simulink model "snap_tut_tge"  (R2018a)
settings: Solver=VariableStepDiscrete  StartTime=0.0  StopTime=50000  RelTol=1e-3
undefined symbols (not defined in the file): bad_frame, Bit, Both, bram, c, cnt_rst, core_rst, d, data, data_in, eof, eof_in, Falling, hex2dec, ip, ip_in, led, led_rx, led_tx, led_up, link_up, Location, Lower, Minimum_Area, notused, out, overrun, reg, Rising, ROACH2, sfp, SNAP, tx_full, tx_over, Unsigned, Upper, valid, valid_in, Width, xc7k160t
libraries: xbsIndex_r4 x1201, casper_library_misc x9, xps_library x5
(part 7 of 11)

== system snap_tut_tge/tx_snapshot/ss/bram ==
  addr : Inport
  data_in : Inport  Port=2
  we : Inport  Port=3
  Terminator : Terminator
  Terminator1 : Terminator
  Terminator2 : Terminator
  calc_add : Subsystem  mask{data_width=128, addr_width=12, sample_rate=sample_rate}
      mask prompts: data_width "data width"; addr_width "address width"; sample_rate "sample rate"
  convert_addr : xbsIndex_r4/Convert  gui_display_data_type=Fixed-point  arith_type=Unsigned  n_bits=addr_width  bin_pt=0  float_type=Single  exp_bits=8  fraction_bits=24  quantization=Truncate  overflow=Wrap  en=off  latency=0  pipeline=off  dbl_ovrd=off  block_type=convert
  convert_din1 : xbsIndex_r4/Convert  gui_display_data_type=Fixed-point  arith_type=Unsigned  n_bits=128  bin_pt=0  float_type=Single  exp_bits=8  fraction_bits=24  quantization=Truncate  overflow=Wrap  en=off  latency=0  pipeline=off  dbl_ovrd=off  block_type=convert
  convert_we : xbsIndex_r4/Convert  gui_display_data_type=Fixed-point  arith_type=Unsigned  n_bits=1  bin_pt=0  float_type=Single  exp_bits=8  fraction_bits=24  quantization=Truncate  overflow=Wrap  en=off  latency=0  pipeline=off  dbl_ovrd=off  block_type=convert
  munge_in : Subsystem  AncestorBlock=casper_library_flow_control/munge  mask(munge){divisions=4, div_size=[32 32 32 32], order=[3  2  1  0], arith_type_out=Unsigned, bin_pt_out=0}
      mask prompts: divisions "Number of divisions"; div_size "Division size (bits)"; order "Division packing order"; arith_type_out "Output arithmetic type"; bin_pt_out "Output binary point"
      mask help: Splits an input bus into the specified number of divisions and then recombines them in the order specified (most significant division = 0,least = number divisions-1)
      mask init:
      | munge_init(gcb, ...
      |     'divisions', divisions, ...
      |     'div_size', div_size, ...
      |     'order', order, ...
      |     'arith_type_out', arith_type_out, ...
      |     'bin_pt_out', bin_pt_out);
  munge_out : Subsystem  AncestorBlock=casper_library_flow_control/munge  mask(munge){divisions=4, div_size=[32 32 32 32], order=[3  2  1  0], arith_type_out=Unsigned, bin_pt_out=0}
      mask prompts: divisions "Number of divisions"; div_size "Division size (bits)"; order "Division packing order"; arith_type_out "Output arithmetic type"; bin_pt_out "Output binary point"
      mask help: Splits an input bus into the specified number of divisions and then recombines them in the order specified (most significant division = 0,least = number divisions-1)
      mask init:
      | munge_init(gcb, ...
      |     'divisions', divisions, ...
      |     'div_size', div_size, ...
      |     'order', order, ...
      |     'arith_type_out', arith_type_out, ...
      |     'bin_pt_out', bin_pt_out);
  sim_mem : Subsystem  mask{arith_type=Unsigned, addr_width=12, data_width=128, data_bin_pt=0, init_vals=[0     1     2     3     4     5     6     7     8     9    10    11    12    13    14    15    16    17    18    19    20    21    22    23    24    25    26    27    28    29    30    31    32    33    34    35    36    37    38    39    40    41    42    43    44    45    46    47    48    49    50    51    52    53    54    55    56    57    58    59    60    61    62    63    64    65    66  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, sample_rate=1, csp_latency=1}
      mask prompts: arith_type "Output Data Type"; addr_width "Address width"; data_width "Data width"; data_bin_pt "Data Binary Point"; init_vals "Initial values"; sample_rate "Sample rate"; csp_latency "Latency"
      mask init:
      | % set_param([gcb, '/data_to_xilinx'], 'arith_type', arith_type)
      | % set_param([gcb, '/data_to_xilinx'], 'n_bits', get_param(gcb, 'data_width'))
  snap_tut_tge_tx_snapshot_ss_bram_addr : xbsIndex_r4/Gateway Out  inherit_from_input=off  hdl_port=on  rows=1  columns=1  UseAsDAC=off  DACChannel='1'  interface=None  automatic_assignment=on  address_offset=hex2dec('00')  intf_name=''  intf_description=''  timing_constraint=None  locs_specified=off  LOCs={'A5','B9','A9','C1','A3','G6','E9','A6','A7','A8','B8','B1','B3','D9','B5','B4','B6','C2'}  io_standard={}  block_type=gatewayout
  snap_tut_tge_tx_snapshot_ss_bram_data_in : xbsIndex_r4/Gateway Out  inherit_from_input=off  hdl_port=on  rows=1  columns=1  UseAsDAC=off  DACChannel='1'  interface=None  automatic_assignment=on  address_offset=hex2dec('00')  intf_name=''  intf_description=''  timing_constraint=None  locs_specified=off  LOCs={'B21','B22','A22','B23','B19','C19','A20','A21','A23','B24','A24','A25','E18','D18','C18','B18'}  io_standard={}  block_type=gatewayout
  snap_tut_tge_tx_snapshot_ss_bram_data_out : xbsIndex_r4/Gateway In  gui_display_data_type=Fixed-point  arith_type=Unsigned  n_bits=128  bin_pt=0  preci_type=Single  exp_width=8  frac_width=24  rows=1  columns=1  quantization=Truncate  overflow=Wrap  period=sample_rate  UseAsADC=off  ADCChannel='1'  interface=None  automatic_assignment=on  address_offset=hex2dec('00')  intf_name=''  intf_description=''  default_value=0  timing_constraint=None  locs_specified=off  LOCs={}  io_standard={}  inherit_from_input=off  hdl_port=on  dbl_ovrd=off  block_type=gatewayin
  snap_tut_tge_tx_snapshot_ss_bram_we : xbsIndex_r4/Gateway Out  inherit_from_input=off  hdl_port=on  rows=1  columns=1  UseAsDAC=off  DACChannel='1'  interface=None  automatic_assignment=on  address_offset=hex2dec('00')  intf_name=''  intf_description=''  timing_constraint=None  locs_specified=off  LOCs={'A14'}  io_standard={}  block_type=gatewayout
  data_out : Outport
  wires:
  munge_in/1(dout) -> convert_din1/1, sim_mem/2(data)
  we/1 -> convert_we/1, sim_mem/3(we)
  addr/1 -> calc_add/1(in)
  convert_we/1 -> snap_tut_tge_tx_snapshot_ss_bram_we/1
  snap_tut_tge_tx_snapshot_ss_bram_addr/1 -> Terminator/1
  snap_tut_tge_tx_snapshot_ss_bram_data_in/1 -> Terminator1/1
  snap_tut_tge_tx_snapshot_ss_bram_we/1 -> Terminator2/1
  calc_add/1(out) -> convert_addr/1, sim_mem/1(addr)
  data_in/1 -> munge_in/1(din)
  convert_din1/1 -> snap_tut_tge_tx_snapshot_ss_bram_data_in/1
  convert_addr/1 -> snap_tut_tge_tx_snapshot_ss_bram_addr/1
  snap_tut_tge_tx_snapshot_ss_bram_data_out/1 -> munge_out/1(din)
  sim_mem/1(data_out) -> snap_tut_tge_tx_snapshot_ss_bram_data_out/1
  munge_out/1(dout) -> data_out/1

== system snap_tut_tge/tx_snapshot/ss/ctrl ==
  convert1_1 : DataTypeConversion  OutDataTypeStr=fixdt('ufix32_En0')
  convert2_1 : DataTypeConversion  OutDataTypeStr=fixdt('ufix32_En0')  ConvertRealWorld=Stored Integer (SI)
  gain_1 : Gain
  io_delay : xbsIndex_r4/Delay  rst=off  infoeditControl=Selection of Reset will increase slice count due to use of real FFs and instead of SRLs  en=off  latency=0  reg_retiming=on  dbl_ovrd=off  block_type=delay
  reint1 : xbsIndex_r4/Reinterpret  force_arith_type=on  arith_type=Unsigned  force_bin_pt=on  bin_pt=0  block_type=reinterpret
  sim_1 : Constant  Value=0
  slice_reg : xbsIndex_r4/Slice  nbits=32  boolean_output=off  mode=Lower Bit Location + Width  bit1=0  base1=MSB of Input  bit0=0  base0=LSB of Input  dbl_ovrd=off  block_type=slice
  snap_tut_tge_tx_snapshot_ss_ctrl_user_data_out : xbsIndex_r4/Gateway In  gui_display_data_type=Fixed-point  arith_type=Unsigned  n_bits=32  bin_pt=0  preci_type=Single  exp_width=8  frac_width=24  rows=1  columns=1  quantization="Round  (unbiased: +/- Inf)"  overflow=Saturate  period=1  UseAsADC=off  ADCChannel='1'  interface=None  automatic_assignment=on  address_offset=hex2dec('00')  intf_name=''  intf_description=''  default_value=0  timing_constraint=None  locs_specified=off  LOCs={}  io_standard={}  inherit_from_input=off  hdl_port=on  dbl_ovrd=off  block_type=gatewayin
  in_reg : Outport
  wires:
  snap_tut_tge_tx_snapshot_ss_ctrl_user_data_out/1 -> io_delay/1
  sim_1/1 -> convert1_1/1
  convert1_1/1 -> convert2_1/1
  convert2_1/1 -> gain_1/1
  gain_1/1 -> snap_tut_tge_tx_snapshot_ss_ctrl_user_data_out/1
  io_delay/1 -> slice_reg/1
  slice_reg/1 -> reint1/1
  reint1/1 -> in_reg/1

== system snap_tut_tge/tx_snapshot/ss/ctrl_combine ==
  in1 : Inport
  in2 : Inport  Port=2
  in3 : Inport  Port=3
  in4 : Inport  Port=4
  concatenate : xbsIndex_r4/Concat  num_inputs=4  dbl_ovrd=off  block_type=concat
  reinterpret{1..4} (4 alike) : xbsIndex_r4/Reinterpret  force_arith_type=on  arith_type=Unsigned  force_bin_pt=on  bin_pt=0  block_type=reinterpret
  bus_out : Outport
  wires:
  concatenate/1 -> bus_out/1
  in1/1 -> reinterpret1/1
  reinterpret1/1 -> concatenate/1
  in2/1 -> reinterpret2/1
  reinterpret2/1 -> concatenate/2
  in3/1 -> reinterpret3/1
  reinterpret3/1 -> concatenate/3
  in4/1 -> reinterpret4/1
  reinterpret4/1 -> concatenate/4

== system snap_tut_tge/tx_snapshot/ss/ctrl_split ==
  bus_in : Inport
  reinterpret2 : xbsIndex_r4/Reinterpret  force_arith_type=on  arith_type=Unsigned  force_bin_pt=on  bin_pt=0  block_type=reinterpret
  reinterpret4 : xbsIndex_r4/Reinterpret  force_arith_type=on  arith_type=Unsigned  force_bin_pt=on  bin_pt=0  block_type=reinterpret
  slice1 : xbsIndex_r4/Slice  nbits=1  boolean_output=on  mode=Upper Bit Location + Width  bit1=-31  base1=MSB of Input  bit0=0  base0=LSB of Input  dbl_ovrd=off  block_type=slice
  slice2 : xbsIndex_r4/Slice  nbits=2  boolean_output=off  mode=Upper Bit Location + Width  bit1=-29  base1=MSB of Input  bit0=0  base0=LSB of Input  dbl_ovrd=off  block_type=slice
  slice3 : xbsIndex_r4/Slice  nbits=1  boolean_output=on  mode=Upper Bit Location + Width  bit1=-28  base1=MSB of Input  bit0=0  base0=LSB of Input  dbl_ovrd=off  block_type=slice
  slice4 : xbsIndex_r4/Slice  nbits=28  boolean_output=off  mode=Upper Bit Location + Width  bit1=0  base1=MSB of Input  bit0=0  base0=LSB of Input  dbl_ovrd=off  block_type=slice
  msb_out4 : Outport
  out3 : Outport  Port=2
  out2 : Outport  Port=3
  lsb_out1 : Outport  Port=4
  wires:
  bus_in/1 -> slice4/1, slice3/1, slice2/1, slice1/1
  slice4/1 -> reinterpret4/1
  reinterpret4/1 -> msb_out4/1
  slice3/1 -> out3/1
  slice2/1 -> reinterpret2/1
  reinterpret2/1 -> out2/1
  slice1/1 -> lsb_out1/1

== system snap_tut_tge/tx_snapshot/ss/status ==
  out_reg : Inport
  assert_reg : xbsIndex_r4/Assert  assert_type=on  type_source=Explicitly  gui_display_data_type=Fixed-point  arith_type=Unsigned  n_bits=32  bin_pt=0  preci_type=Single  exp_width=8  frac_width=24  assert_rate=off  rate_source=Explicitly  period=1  output_port=on  block_type=assert
  cast_gw : xbsIndex_r4/Convert  gui_display_data_type=Fixed-point  arith_type=Unsigned  n_bits=32  bin_pt=0  float_type=Single  exp_bits=8  fraction_bits=24  quantization=Truncate  overflow=Wrap  en=off  latency=1  pipeline=off  dbl_ovrd=off  block_type=convert
  io_delay : xbsIndex_r4/Delay  rst=off  infoeditControl=Selection of Reset will increase slice count due to use of real FFs and instead of SRLs  en=off  latency=0  reg_retiming=on  dbl_ovrd=off  block_type=delay
  reint1 : xbsIndex_r4/Reinterpret  force_arith_type=on  arith_type=Unsigned  force_bin_pt=on  bin_pt=0  block_type=reinterpret
  sim_out : Terminator
  snap_tut_tge_tx_snapshot_ss_status_user_data_in : xbsIndex_r4/Gateway Out  inherit_from_input=off  hdl_port=on  rows=1  columns=1  UseAsDAC=off  DACChannel='1'  interface=None  automatic_assignment=on  address_offset=hex2dec('00')  intf_name=''  intf_description=''  timing_constraint=None  locs_specified=off  LOCs={}  io_standard={}  block_type=gatewayout
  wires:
  io_delay/1 -> cast_gw/1
  cast_gw/1 -> snap_tut_tge_tx_snapshot_ss_status_user_data_in/1
  snap_tut_tge_tx_snapshot_ss_status_user_data_in/1 -> sim_out/1
  out_reg/1 -> assert_reg/1
  assert_reg/1 -> reint1/1
  reint1/1 -> io_delay/1

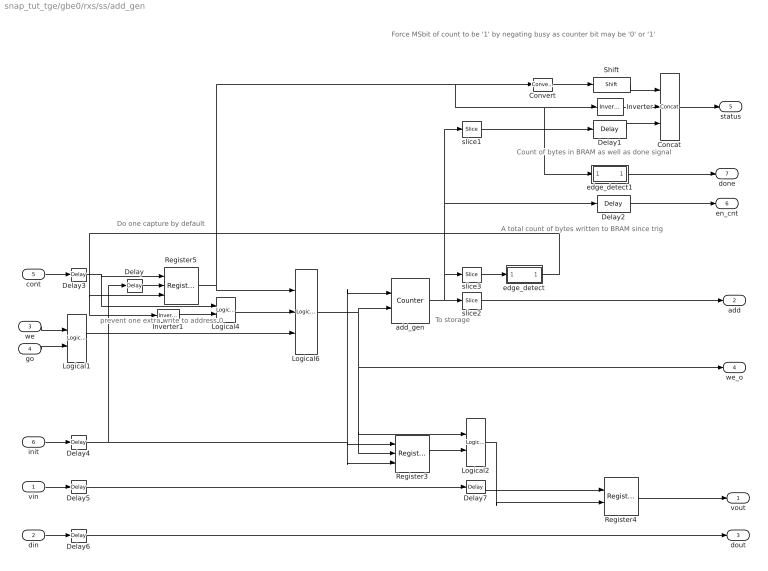
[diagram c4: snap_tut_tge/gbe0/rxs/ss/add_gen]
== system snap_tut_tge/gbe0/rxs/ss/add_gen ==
  note: Force MSbit of count to be '1' by negating busy as counter bit may be '0' or '1'
  note: A total count of bytes written to BRAM since trig
  note: Count of bytes in BRAM as well as done signal
  note: Do one capture by default
  note: prevent one extra write to address 0
  note: To storage
  vin : Inport
  din : Inport  Port=2
  we : Inport  Port=3
  go : Inport  Port=4
  cont : Inport  Port=5
  init : Inport  Port=6
  Concat : xbsIndex_r4/Concat  num_inputs=3  dbl_ovrd=off  block_type=concat
  Convert : xbsIndex_r4/Convert  gui_display_data_type=Fixed-point  arith_type=Unsigned  n_bits=32-nsamples-log2(increment)-1  bin_pt=0  float_type=Single  exp_bits=8  fraction_bits=24  quantization=Truncate  overflow=Wrap  en=off  latency=0  pipeline=off  dbl_ovrd=off  block_type=convert
  Delay{,3..6} (5 alike) : xbsIndex_r4/Delay  rst=off  infoeditControl=Selection of Reset will increase slice count due to use of real FFs and instead of SRLs  en=off  latency=1  reg_retiming=on  dbl_ovrd=off  block_type=delay
  Delay1 : xbsIndex_r4/Delay  rst=off  infoeditControl=Selection of Reset will increase slice count due to use of real FFs and instead of SRLs  en=off  latency=1  reg_retiming=off  dbl_ovrd=off  block_type=delay
  Delay2 : xbsIndex_r4/Delay  rst=off  infoeditControl=Selection of Reset will increase slice count due to use of real FFs and instead of SRLs  en=off  latency=1  reg_retiming=off  dbl_ovrd=off  block_type=delay
  Delay7 : xbsIndex_r4/Delay  rst=off  infoeditControl=Selection of Reset will increase slice count due to use of real FFs and instead of SRLs  en=off  latency=1  reg_retiming=off  dbl_ovrd=off  block_type=delay
  Inverter : xbsIndex_r4/Inverter  en=off  latency=1  dbl_ovrd=off  block_type=inv
  Inverter1 : xbsIndex_r4/Inverter  en=off  latency=0  dbl_ovrd=off  block_type=inv
  Logical1 : xbsIndex_r4/Logical  logical_function=AND  inputs=2  en=off  latency=1  precision=Full  arith_type=Unsigned  n_bits=8  bin_pt=2  align_bp=on  dbl_ovrd=off  block_type=logical
  Logical2 : xbsIndex_r4/Logical  logical_function=AND  inputs=2  en=off  latency=1  precision=Full  arith_type=Unsigned  n_bits=8  bin_pt=2  align_bp=on  dbl_ovrd=off  block_type=logical
  Logical4 : xbsIndex_r4/Logical  logical_function=OR  inputs=2  en=off  latency=0  precision=Full  arith_type=Unsigned  n_bits=8  bin_pt=2  align_bp=on  dbl_ovrd=off  block_type=logical
  Logical6 : xbsIndex_r4/Logical  logical_function=AND  inputs=3  en=off  latency=0  precision=Full  arith_type=Unsigned  n_bits=8  bin_pt=2  align_bp=on  dbl_ovrd=off  block_type=logical
  Register3 : xbsIndex_r4/Register  init=0  rst=on  en=on  dbl_ovrd=off  block_type=register
  Register4 : xbsIndex_r4/Register  init=0  rst=off  en=on  dbl_ovrd=off  block_type=register
  Register5 : xbsIndex_r4/Register  init=1  rst=on  en=on  dbl_ovrd=off  block_type=register
  Shift : xbsIndex_r4/Shift  shift_dir=Left  shift_bits=32-nsamples-log2(increment)-1-1  en=off  latency=1  precision=Full  arith_type="Signed  (2's comp)"  n_bits=16  bin_pt=14  quantization=Truncate  overflow=Wrap  dbl_ovrd=off  block_type=shift
  add_gen : xbsIndex_r4/Counter  cnt_type=Free Running  cnt_to=1  operation=Up  start_count=0  cnt_by_val=increment  arith_type=Unsigned  n_bits=counter_size  bin_pt=0  load_pin=off  rst=on  en=on  explicit_period=on  period=1  use_behavioral_HDL=off  implementation=DSP48  use_rpm=on  dbl_ovrd=off  block_type=counter
  edge_detect : Subsystem  AncestorBlock=casper_library_misc/edge_detect  mask(edge_detect){edge=Both, polarity=Active High, x_in=[0 0.08 0.08 0.16 0.16 0.24 0.24 0.32 0.32 0.4], y_in=[-1 -1  1  1  1  1 -1 -1 -1 -1], x_out=[0.6 0.68 0.68 0.76 0.76 0.84 0.84 0.92 0.92 1], y_out=[-1 -1  1  1 -1 -1  1  1 -1 -1]}
      mask prompts: edge "Edge Type"; polarity "Output Polarity"; x_in "Input X Positions"; y_in "Input Y Positions"; x_out "Output X Positions"; y_out "Output Y Positions"
      mask help: Output is active for one-cycle after each edge of the specified type (i.e. rising, falling or both).
      mask init:
      | edge_detect_init(gcb,...
      |     'edge',edge,...
      |     'polarity',polarity,...
      |     'x_in',x_in,...
      |     'x_out',x_out,...
      |     'y_in',y_in,...
      |     'y_out',y_out);
      | 
      | x_in_num=str2num(getfield(getfield(get_param(gcb,'UserData'),'parameters'),'x_in'));
      | x_out_num=str2num(getfield(getfield(get_param(gcb,'UserData'),'parameters'),'x_out'));
      | y_in_num=str2num(getfield(getfield(get_param(gcb,'UserData'),'parameters'),'y_in'));
      | y_out_num=str2num(getfield(getfield(get_param(gcb,'UserData'),'parameters'),'y_out'));
  edge_detect1 : Subsystem  AncestorBlock=casper_library_scopes/snapshot/add_gen/edge_detect  mask(edge_detect){edge=Both, polarity=Active High, x_in=[0 0.08 0.08 0.16 0.16 0.24 0.24 0.32 0.32 0.4], y_in=[-1 -1  1  1  1  1 -1 -1 -1 -1], x_out=[0.6 0.68 0.68 0.76 0.76 0.84 0.84 0.92 0.92 1], y_out=[-1 -1  1  1 -1 -1  1  1 -1 -1]}
      mask prompts: edge "Edge Type"; polarity "Output Polarity"; x_in "Input X Positions"; y_in "Input Y Positions"; x_out "Output X Positions"; y_out "Output Y Positions"
      mask help: Output is active for one-cycle after each edge of the specified type (i.e. rising, falling or both).
      mask init:
      | edge_detect_init(gcb,...
      |     'edge',edge,...
      |     'polarity',polarity,...
      |     'x_in',x_in,...
      |     'x_out',x_out,...
      |     'y_in',y_in,...
      |     'y_out',y_out);
      | 
      | x_in_num=str2num(getfield(getfield(get_param(gcb,'UserData'),'parameters'),'x_in'));
      | x_out_num=str2num(getfield(getfield(get_param(gcb,'UserData'),'parameters'),'x_out'));
      | y_in_num=str2num(getfield(getfield(get_param(gcb,'UserData'),'parameters'),'y_in'));
      | y_out_num=str2num(getfield(getfield(get_param(gcb,'UserData'),'parameters'),'y_out'));
  slice1 : xbsIndex_r4/Slice  nbits=nsamples+log2(increment)  boolean_output=off  mode=Lower Bit Location + Width  bit1=0  base1=LSB of Input  bit0=0  base0=LSB of Input  dbl_ovrd=off  block_type=slice
  slice2 : xbsIndex_r4/Slice  nbits=nsamples-burst_size  boolean_output=off  mode=Lower Bit Location + Width  bit1=0  base1=LSB of Input  bit0=log2(increment)+burst_size  base0=LSB of Input  dbl_ovrd=off  block_type=slice
  slice3 : xbsIndex_r4/Slice  nbits=1  boolean_output=on  mode=Lower Bit Location + Width  bit1=0  base1=MSB of Input  bit0=nsamples + log2(increment)  base0=LSB of Input  dbl_ovrd=off  block_type=slice
  vout : Outport
  add : Outport  Port=2
  dout : Outport  Port=3
  we_o : Outport  Port=4
  status : Outport  Port=5
  en_cnt : Outport  Port=6
  done : Outport  Port=7
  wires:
  Delay6/1 -> dout/1
  Delay5/1 -> Delay7/1
  Delay4/1 -> Delay/1, Register3/1, Register3/3, add_gen/1
  Delay3/1 -> Register5/1, Logical4/1
  Delay7/1 -> Register4/1
  Logical1/1 -> Logical6/3
  go/1 -> Logical1/2
  we/1 -> Logical1/1
  Logical4/1 -> Logical6/2
  Inverter/1 -> Concat/2
  slice1/1 -> Delay1/1
  Delay1/1 -> Concat/3
  din/1 -> Delay6/1
  Delay2/1 -> en_cnt/1
  slice2/1 -> add/1
  Convert/1 -> Shift/1
  Concat/1 -> status/1
  Logical6/1 -> add_gen/2, Register3/2, Logical2/1, we_o/1
  init/1 -> Delay4/1
  slice3/1 -> edge_detect/1(in)
  Register5/1 -> Logical6/1, edge_detect1/1(in), Inverter/1, Convert/1
  add_gen/1 -> slice3/1, Delay2/1, slice1/1, slice2/1
  vin/1 -> Delay5/1
  Register3/1 -> Logical2/2
  Logical2/1 -> Register4/2
  Register4/1 -> vout/1
  edge_detect/1(out) -> Register5/3, Inverter1/1
  cont/1 -> Delay3/1
  Inverter1/1 -> Logical4/2
  Delay/1 -> Register5/2
  Shift/1 -> Concat/1
  edge_detect1/1(out) -> done/1

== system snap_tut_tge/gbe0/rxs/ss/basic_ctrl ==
  vin : Inport
  din : Inport  Port=2
  we : Inport  Port=3
  trig : Inport  Port=4
  ctrl : Inport  Port=5
  stopi : Inport  Port=6
  Constant : xbsIndex_r4/Constant  const=1  gui_display_data_type=Fixed-point  arith_type=Boolean  n_bits=16  bin_pt=14  preci_type=Single  exp_width=8  frac_width=24  explicit_period=on  period=1  equ=P=C  opselect=C  inp2=PCIN>>17  opr=+  inp1=P  carry=CIN  dbl_ovrd=off  block_type=constant
  Constant1 : xbsIndex_r4/Constant  const=1  gui_display_data_type=Fixed-point  arith_type=Boolean  n_bits=1  bin_pt=0  preci_type=Single  exp_width=8  frac_width=24  explicit_period=on  period=1  equ=P=C  opselect=C  inp2=PCIN>>17  opr=+  inp1=P  carry=CIN  dbl_ovrd=off  block_type=constant
  Constant2 : xbsIndex_r4/Constant  const=1  gui_display_data_type=Fixed-point  arith_type=Boolean  n_bits=1  bin_pt=0  preci_type=Single  exp_width=8  frac_width=24  explicit_period=on  period=1  equ=P=C  opselect=C  inp2=PCIN>>17  opr=+  inp1=P  carry=CIN  dbl_ovrd=off  block_type=constant
  Delay1 : xbsIndex_r4/Delay  rst=off  infoeditControl=Selection of Reset will increase slice count due to use of real FFs and instead of SRLs  en=off  latency=1  reg_retiming=off  dbl_ovrd=off  block_type=delay
  Delay2 : xbsIndex_r4/Delay  rst=off  infoeditControl=Selection of Reset will increase slice count due to use of real FFs and instead of SRLs  en=off  latency=1  reg_retiming=off  dbl_ovrd=off  block_type=delay
  Delay3 : xbsIndex_r4/Delay  rst=off  infoeditControl=Selection of Reset will increase slice count due to use of real FFs and instead of SRLs  en=off  latency=1  reg_retiming=off  dbl_ovrd=off  block_type=delay
  Inverter : xbsIndex_r4/Inverter  en=off  latency=0  dbl_ovrd=off  block_type=inv
  Logical : xbsIndex_r4/Logical  logical_function=AND  inputs=2  en=off  latency=0  precision=Full  arith_type=Unsigned  n_bits=16  bin_pt=0  align_bp=on  dbl_ovrd=off  block_type=logical
  Mux1 : xbsIndex_r4/Mux  inputs=2  en=off  latency=0  precision=Full  arith_type="Signed  (2's comp)"  n_bits=8  bin_pt=2  quantization=Truncate  overflow=Wrap  dbl_ovrd=off  block_type=mux
  Mux2 : xbsIndex_r4/Mux  inputs=2  en=off  latency=0  precision=Full  arith_type="Signed  (2's comp)"  n_bits=8  bin_pt=2  quantization=Truncate  overflow=Wrap  dbl_ovrd=off  block_type=mux
  Register1 : xbsIndex_r4/Register  init=0  rst=on  en=on  dbl_ovrd=off  block_type=register
  Register6 : xbsIndex_r4/Register  init=0  rst=on  en=on  dbl_ovrd=off  block_type=register
  dram_munge : Subsystem  mask{dram=off, data_width=data_width}
      mask prompts: data_width "data width"
      mask init:
      | set_param(gcb,'LinkStatus','inactive');
      | if strcmp(dram,'on'),
      |     set_param([gcb,'/dram'], 'const', '1');
      | else,
      |     set_param([gcb,'/dram'], 'const', '0');
      | end
      | set_param([gcb,'/data_choice'], ...
      |         'precision', 'User Defined', ...
      |         'arith_type', 'Unsigned', ...
      |         'n_bits', num2str(data_width), 'bin_pt', '0', ...
      |         'quantization', 'Truncate', ...
      |         'overflow', 'Wrap');
  edge_detect : casper_library_misc/edge_detect  edge=Rising  polarity=Active High  x_in=[0 0.08 0.08 0.16 0.16 0.24 0.24 0.32 0.32 0.4]  y_in="[-1 -1  1  1  1  1  1  1  1  1]"  x_out=[0.6 0.68 0.68 0.76 0.76 0.84 0.84 0.92 0.92 1]  y_out="[-1 -1  1  1 -1 -1 -1 -1 -1 -1]"
      link override Delay: sg_icon_stat=45,16,1,1,white,blue,0,07b98262,right,,[ ],[ ]  sg_mask_display=fprintf('','COMMENT: begin icon graphics'); patch([0 45 45 0 0 ],[0 0 16 16 0 ],[0.77 0.82 0.91 ]); plot([0 45 45 0 0 ],[0 0 16 16 0 ]); patch([17.55 20.44 22.44 24.44 26.44 22.44 19.55 17.55 ],[10.22 10.22 12.22 10.22 12.22 12.22 12.22 10.22 ],[1 1 1 ]); patch([19.55 22.44 20.44 17.55 19.55 ],[8.22 8.22 10.22 10.22 8.22 ],[0.931 0.946 0.973 ]); patch([17.55 20.44 22.44 19.55 17.55 ],[6.22 6.22 8.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
      link override Inverter: sg_icon_stat=45,16,1,1,white,blue,0,267846e5,right,,[ ],[ ]  sg_mask_display=fprintf('','COMMENT: begin icon graphics'); patch([0 45 45 0 0 ],[0 0 16 16 0 ],[0.77 0.82 0.91 ]); plot([0 45 45 0 0 ],[0 0 16 16 0 ]); patch([17.55 20.44 22.44 24.44 26.44 22.44 19.55 17.55 ],[10.22 10.22 12.22 10.22 12.22 12.22 12.22 10.22 ],[1 1 1 ]); patch([19.55 22.44 20.44 17.55 19.55 ],[8.22 8.22 10.22 10.22 8.22 ],[0.931 0.946 0.973 ]); patch([17.55 20.44 22.44 19.55 17.55 ],[6.22 6.22 8.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
      link override edge_op: sg_icon_stat=45,44,2,1,white,blue,0,affe8783,right,,[ ],[ ]  sg_mask_display=fprintf('','COMMENT: begin icon graphics'); patch([0 45 45 0 0 ],[0 0 44 44 0 ],[0.77 0.82 0.91 ]); plot([0 45 45 0 0 ],[0 0 44 44 0 ]); patch([8.65 17.32 23.32 29.32 35.32 23.32 14.65 8.65 ],[28.66 28.66 34.66 28.66 34.66 34.66 34.66 28.66 ],[1 1 1 ]); patch([14.65 23.32 17.32 8.65 14.65 ],[22.66 22.66 28.66 28.66 22.66 ],[0.931 0.946 0.973 ]); patch([8.65 17.32 23.32 14.65 8.65 ],[16.66 16.66 22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
  enable : xbsIndex_r4/Slice  nbits=1  boolean_output=on  mode=Lower Bit Location + Width  bit1=0  base1=LSB of Input  bit0=0  base0=LSB of Input  dbl_ovrd=off  block_type=slice
  trig_src : xbsIndex_r4/Slice  nbits=1  boolean_output=on  mode=Lower Bit Location + Width  bit1=0  base1=LSB of Input  bit0=1  base0=LSB of Input  dbl_ovrd=off  block_type=slice
  valid_src : xbsIndex_r4/Slice  nbits=1  boolean_output=on  mode=Lower Bit Location + Width  bit1=0  base1=LSB of Input  bit0=2  base0=LSB of Input  dbl_ovrd=off  block_type=slice
  vout : Outport
  dout : Outport  Port=2
  we_o : Outport  Port=3
  go : Outport  Port=4
  stop : Outport  Port=5
  init : Outport  Port=6
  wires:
  Delay1/1 -> edge_detect/1
  Delay3/1 -> Mux1/1
  Delay2/1 -> Mux2/1
  dram_munge/1(vout) -> vout/1
  vin/1 -> dram_munge/1(vin)
  dram_munge/3(we_o) -> we_o/1
  dram_munge/2(dout) -> dout/1
  din/1 -> dram_munge/2(din)
  Inverter/1 -> Logical/2
  Mux2/1 -> Logical/1, Register6/1
  Register6/1 -> go/1
  trig/1 -> Mux2/2
  Mux1/1 -> dram_munge/3(we)
  we/1 -> Mux1/2
  ctrl/1 -> enable/1, valid_src/1, trig_src/1
  edge_detect/1 -> Inverter/1, Register1/3, dram_munge/4(init), Register6/2, init/1
  enable/1 -> Delay1/1
  Constant1/1 -> Mux2/3
  Constant2/1 -> Mux1/3
  trig_src/1 -> Delay2/1
  valid_src/1 -> Delay3/1
  Constant/1 -> Register1/1
  Register1/1 -> Register6/3
  Logical/1 -> Register1/2
  stopi/1 -> stop/1

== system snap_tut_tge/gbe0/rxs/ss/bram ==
  addr : Inport
  data_in : Inport  Port=2
  we : Inport  Port=3
  Terminator : Terminator
  Terminator1 : Terminator
  Terminator2 : Terminator
  calc_add : Subsystem  mask{data_width=128, addr_width=13, sample_rate=sample_rate}
      mask prompts: data_width "data width"; addr_width "address width"; sample_rate "sample rate"
  convert_addr : xbsIndex_r4/Convert  gui_display_data_type=Fixed-point  arith_type=Unsigned  n_bits=addr_width  bin_pt=0  float_type=Single  exp_bits=8  fraction_bits=24  quantization=Truncate  overflow=Wrap  en=off  latency=0  pipeline=off  dbl_ovrd=off  block_type=convert
  convert_din1 : xbsIndex_r4/Convert  gui_display_data_type=Fixed-point  arith_type=Unsigned  n_bits=128  bin_pt=0  float_type=Single  exp_bits=8  fraction_bits=24  quantization=Truncate  overflow=Wrap  en=off  latency=0  pipeline=off  dbl_ovrd=off  block_type=convert
  convert_we : xbsIndex_r4/Convert  gui_display_data_type=Fixed-point  arith_type=Unsigned  n_bits=1  bin_pt=0  float_type=Single  exp_bits=8  fraction_bits=24  quantization=Truncate  overflow=Wrap  en=off  latency=0  pipeline=off  dbl_ovrd=off  block_type=convert
  munge_in : Subsystem  AncestorBlock=casper_library_flow_control/munge  mask(munge){divisions=4, div_size=[32 32 32 32], order=[3  2  1  0], arith_type_out=Unsigned, bin_pt_out=0}
      mask prompts: divisions "Number of divisions"; div_size "Division size (bits)"; order "Division packing order"; arith_type_out "Output arithmetic type"; bin_pt_out "Output binary point"
      mask help: Splits an input bus into the specified number of divisions and then recombines them in the order specified (most significant division = 0,least = number divisions-1)
      mask init:
      | munge_init(gcb, ...
      |     'divisions', divisions, ...
      |     'div_size', div_size, ...
      |     'order', order, ...
      |     'arith_type_out', arith_type_out, ...
      |     'bin_pt_out', bin_pt_out);
  munge_out : Subsystem  AncestorBlock=casper_library_flow_control/munge  mask(munge){divisions=4, div_size=[32 32 32 32], order=[3  2  1  0], arith_type_out=Unsigned, bin_pt_out=0}
      mask prompts: divisions "Number of divisions"; div_size "Division size (bits)"; order "Division packing order"; arith_type_out "Output arithmetic type"; bin_pt_out "Output binary point"
      mask help: Splits an input bus into the specified number of divisions and then recombines them in the order specified (most significant division = 0,least = number divisions-1)
      mask init:
      | munge_init(gcb, ...
      |     'divisions', divisions, ...
      |     'div_size', div_size, ...
      |     'order', order, ...
      |     'arith_type_out', arith_type_out, ...
      |     'bin_pt_out', bin_pt_out);
  sim_mem : Subsystem  mask{arith_type=Unsigned, addr_width=13, data_width=128, data_bin_pt=0, init_vals=[0     1     2     3     4     5     6     7     8     9    10    11    12    13    14    15    16    17    18    19    20    21    22    23    24    25    26    27    28    29    30    31    32    33    34    35    36    37    38    39    40    41    42    43    44    45    46    47    48    49    50    51    52    53    54    55    56    57    58    59    60    61    62    63    64    65    66  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, sample_rate=1, csp_latency=1}
      mask prompts: arith_type "Output Data Type"; addr_width "Address width"; data_width "Data width"; data_bin_pt "Data Binary Point"; init_vals "Initial values"; sample_rate "Sample rate"; csp_latency "Latency"
      mask init:
      | % set_param([gcb, '/data_to_xilinx'], 'arith_type', arith_type)
      | % set_param([gcb, '/data_to_xilinx'], 'n_bits', get_param(gcb, 'data_width'))
  snap_tut_tge_gbe0_rxs_ss_bram_addr : xbsIndex_r4/Gateway Out  inherit_from_input=off  hdl_port=on  rows=1  columns=1  UseAsDAC=off  DACChannel='1'  interface=None  automatic_assignment=on  address_offset=hex2dec('00')  intf_name=''  intf_description=''  timing_constraint=None  locs_specified=off  LOCs={'A5','B9','A9','C1','A3','G6','E9','A6','A7','A8','B8','B1','B3','D9','B5','B4','B6','C2'}  io_standard={}  block_type=gatewayout
  snap_tut_tge_gbe0_rxs_ss_bram_data_in : xbsIndex_r4/Gateway Out  inherit_from_input=off  hdl_port=on  rows=1  columns=1  UseAsDAC=off  DACChannel='1'  interface=None  automatic_assignment=on  address_offset=hex2dec('00')  intf_name=''  intf_description=''  timing_constraint=None  locs_specified=off  LOCs={'B21','B22','A22','B23','B19','C19','A20','A21','A23','B24','A24','A25','E18','D18','C18','B18'}  io_standard={}  block_type=gatewayout
  snap_tut_tge_gbe0_rxs_ss_bram_data_out : xbsIndex_r4/Gateway In  gui_display_data_type=Fixed-point  arith_type=Unsigned  n_bits=128  bin_pt=0  preci_type=Single  exp_width=8  frac_width=24  rows=1  columns=1  quantization=Truncate  overflow=Wrap  period=sample_rate  UseAsADC=off  ADCChannel='1'  interface=None  automatic_assignment=on  address_offset=hex2dec('00')  intf_name=''  intf_description=''  default_value=0  timing_constraint=None  locs_specified=off  LOCs={}  io_standard={}  inherit_from_input=off  hdl_port=on  dbl_ovrd=off  block_type=gatewayin
  snap_tut_tge_gbe0_rxs_ss_bram_we : xbsIndex_r4/Gateway Out  inherit_from_input=off  hdl_port=on  rows=1  columns=1  UseAsDAC=off  DACChannel='1'  interface=None  automatic_assignment=on  address_offset=hex2dec('00')  intf_name=''  intf_description=''  timing_constraint=None  locs_specified=off  LOCs={'A14'}  io_standard={}  block_type=gatewayout
  data_out : Outport
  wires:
  munge_in/1(dout) -> convert_din1/1, sim_mem/2(data)
  we/1 -> convert_we/1, sim_mem/3(we)
  addr/1 -> calc_add/1(in)
  convert_we/1 -> snap_tut_tge_gbe0_rxs_ss_bram_we/1
  snap_tut_tge_gbe0_rxs_ss_bram_addr/1 -> Terminator/1
  snap_tut_tge_gbe0_rxs_ss_bram_data_in/1 -> Terminator1/1
  snap_tut_tge_gbe0_rxs_ss_bram_we/1 -> Terminator2/1
  calc_add/1(out) -> convert_addr/1, sim_mem/1(addr)
  data_in/1 -> munge_in/1(din)
  convert_din1/1 -> snap_tut_tge_gbe0_rxs_ss_bram_data_in/1
  convert_addr/1 -> snap_tut_tge_gbe0_rxs_ss_bram_addr/1
  snap_tut_tge_gbe0_rxs_ss_bram_data_out/1 -> munge_out/1(din)
  sim_mem/1(data_out) -> snap_tut_tge_gbe0_rxs_ss_bram_data_out/1
  munge_out/1(dout) -> data_out/1

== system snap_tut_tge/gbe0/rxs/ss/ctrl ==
  convert1_1 : DataTypeConversion  OutDataTypeStr=fixdt('ufix32_En0')
  convert2_1 : DataTypeConversion  OutDataTypeStr=fixdt('ufix32_En0')  ConvertRealWorld=Stored Integer (SI)
  gain_1 : Gain
  io_delay : xbsIndex_r4/Delay  rst=off  infoeditControl=Selection of Reset will increase slice count due to use of real FFs and instead of SRLs  en=off  latency=0  reg_retiming=on  dbl_ovrd=off  block_type=delay
  reint1 : xbsIndex_r4/Reinterpret  force_arith_type=on  arith_type=Unsigned  force_bin_pt=on  bin_pt=0  block_type=reinterpret
  sim_1 : Constant  Value=0
  slice_reg : xbsIndex_r4/Slice  nbits=32  boolean_output=off  mode=Lower Bit Location + Width  bit1=0  base1=MSB of Input  bit0=0  base0=LSB of Input  dbl_ovrd=off  block_type=slice
  snap_tut_tge_gbe0_rxs_ss_ctrl_user_data_out : xbsIndex_r4/Gateway In  gui_display_data_type=Fixed-point  arith_type=Unsigned  n_bits=32  bin_pt=0  preci_type=Single  exp_width=8  frac_width=24  rows=1  columns=1  quantization="Round  (unbiased: +/- Inf)"  overflow=Saturate  period=1  UseAsADC=off  ADCChannel='1'  interface=None  automatic_assignment=on  address_offset=hex2dec('00')  intf_name=''  intf_description=''  default_value=0  timing_constraint=None  locs_specified=off  LOCs={}  io_standard={}  inherit_from_input=off  hdl_port=on  dbl_ovrd=off  block_type=gatewayin
  in_reg : Outport
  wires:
  snap_tut_tge_gbe0_rxs_ss_ctrl_user_data_out/1 -> io_delay/1
  sim_1/1 -> convert1_1/1
  convert1_1/1 -> convert2_1/1
  convert2_1/1 -> gain_1/1
  gain_1/1 -> snap_tut_tge_gbe0_rxs_ss_ctrl_user_data_out/1
  io_delay/1 -> slice_reg/1
  slice_reg/1 -> reint1/1
  reint1/1 -> in_reg/1

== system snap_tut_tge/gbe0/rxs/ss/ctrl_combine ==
  in1 : Inport
  in2 : Inport  Port=2
  in3 : Inport  Port=3
  in4 : Inport  Port=4
  concatenate : xbsIndex_r4/Concat  num_inputs=4  dbl_ovrd=off  block_type=concat
  reinterpret{1..4} (4 alike) : xbsIndex_r4/Reinterpret  force_arith_type=on  arith_type=Unsigned  force_bin_pt=on  bin_pt=0  block_type=reinterpret
  bus_out : Outport
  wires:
  concatenate/1 -> bus_out/1
  in1/1 -> reinterpret1/1
  reinterpret1/1 -> concatenate/1
  in2/1 -> reinterpret2/1
  reinterpret2/1 -> concatenate/2
  in3/1 -> reinterpret3/1
  reinterpret3/1 -> concatenate/3
  in4/1 -> reinterpret4/1
  reinterpret4/1 -> concatenate/4

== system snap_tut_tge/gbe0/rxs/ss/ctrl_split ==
  bus_in : Inport
  reinterpret2 : xbsIndex_r4/Reinterpret  force_arith_type=on  arith_type=Unsigned  force_bin_pt=on  bin_pt=0  block_type=reinterpret
  reinterpret4 : xbsIndex_r4/Reinterpret  force_arith_type=on  arith_type=Unsigned  force_bin_pt=on  bin_pt=0  block_type=reinterpret
  slice1 : xbsIndex_r4/Slice  nbits=1  boolean_output=on  mode=Upper Bit Location + Width  bit1=-31  base1=MSB of Input  bit0=0  base0=LSB of Input  dbl_ovrd=off  block_type=slice
  slice2 : xbsIndex_r4/Slice  nbits=2  boolean_output=off  mode=Upper Bit Location + Width  bit1=-29  base1=MSB of Input  bit0=0  base0=LSB of Input  dbl_ovrd=off  block_type=slice
  slice3 : xbsIndex_r4/Slice  nbits=1  boolean_output=on  mode=Upper Bit Location + Width  bit1=-28  base1=MSB of Input  bit0=0  base0=LSB of Input  dbl_ovrd=off  block_type=slice
  slice4 : xbsIndex_r4/Slice  nbits=28  boolean_output=off  mode=Upper Bit Location + Width  bit1=0  base1=MSB of Input  bit0=0  base0=LSB of Input  dbl_ovrd=off  block_type=slice
  msb_out4 : Outport
  out3 : Outport  Port=2
  out2 : Outport  Port=3
  lsb_out1 : Outport  Port=4
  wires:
  bus_in/1 -> slice4/1, slice3/1, slice2/1, slice1/1
  slice4/1 -> reinterpret4/1
  reinterpret4/1 -> msb_out4/1
  slice3/1 -> out3/1
  slice2/1 -> reinterpret2/1
  reinterpret2/1 -> out2/1
  slice1/1 -> lsb_out1/1

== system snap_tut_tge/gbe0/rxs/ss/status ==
  out_reg : Inport
  assert_reg : xbsIndex_r4/Assert  assert_type=on  type_source=Explicitly  gui_display_data_type=Fixed-point  arith_type=Unsigned  n_bits=32  bin_pt=0  preci_type=Single  exp_width=8  frac_width=24  assert_rate=off  rate_source=Explicitly  period=1  output_port=on  block_type=assert
  cast_gw : xbsIndex_r4/Convert  gui_display_data_type=Fixed-point  arith_type=Unsigned  n_bits=32  bin_pt=0  float_type=Single  exp_bits=8  fraction_bits=24  quantization=Truncate  overflow=Wrap  en=off  latency=1  pipeline=off  dbl_ovrd=off  block_type=convert
  io_delay : xbsIndex_r4/Delay  rst=off  infoeditControl=Selection of Reset will increase slice count due to use of real FFs and instead of SRLs  en=off  latency=0  reg_retiming=on  dbl_ovrd=off  block_type=delay
  reint1 : xbsIndex_r4/Reinterpret  force_arith_type=on  arith_type=Unsigned  force_bin_pt=on  bin_pt=0  block_type=reinterpret
  sim_out : Terminator
  snap_tut_tge_gbe0_rxs_ss_status_user_data_in : xbsIndex_r4/Gateway Out  inherit_from_input=off  hdl_port=on  rows=1  columns=1  UseAsDAC=off  DACChannel='1'  interface=None  automatic_assignment=on  address_offset=hex2dec('00')  intf_name=''  intf_description=''  timing_constraint=None  locs_specified=off  LOCs={}  io_standard={}  block_type=gatewayout
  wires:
  io_delay/1 -> cast_gw/1
  cast_gw/1 -> snap_tut_tge_gbe0_rxs_ss_status_user_data_in/1
  snap_tut_tge_gbe0_rxs_ss_status_user_data_in/1 -> sim_out/1
  out_reg/1 -> assert_reg/1
  assert_reg/1 -> reint1/1
  reint1/1 -> io_delay/1

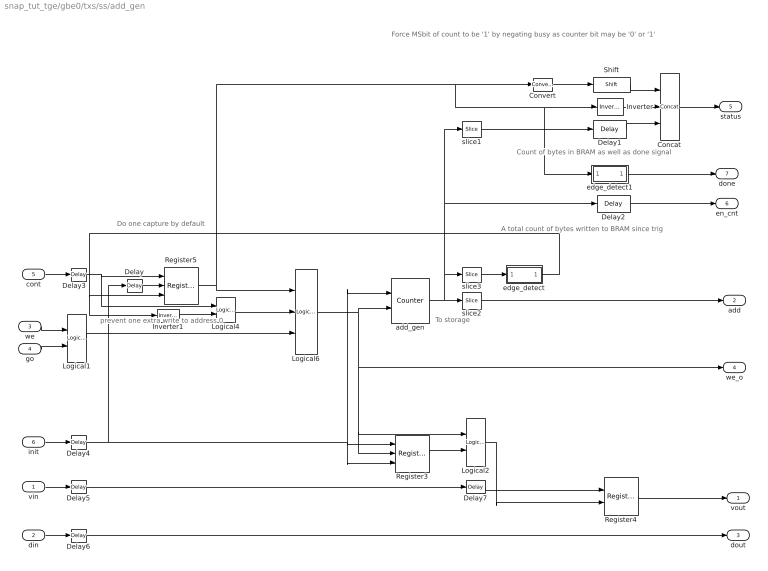
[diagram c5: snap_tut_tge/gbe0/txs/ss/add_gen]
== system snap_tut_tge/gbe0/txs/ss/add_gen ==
  note: Force MSbit of count to be '1' by negating busy as counter bit may be '0' or '1'
  note: A total count of bytes written to BRAM since trig
  note: Count of bytes in BRAM as well as done signal
  note: Do one capture by default
  note: prevent one extra write to address 0
  note: To storage
  vin : Inport
  din : Inport  Port=2
  we : Inport  Port=3
  go : Inport  Port=4
  cont : Inport  Port=5
  init : Inport  Port=6
  Concat : xbsIndex_r4/Concat  num_inputs=3  dbl_ovrd=off  block_type=concat
  Convert : xbsIndex_r4/Convert  gui_display_data_type=Fixed-point  arith_type=Unsigned  n_bits=32-nsamples-log2(increment)-1  bin_pt=0  float_type=Single  exp_bits=8  fraction_bits=24  quantization=Truncate  overflow=Wrap  en=off  latency=0  pipeline=off  dbl_ovrd=off  block_type=convert
  Delay{,3..6} (5 alike) : xbsIndex_r4/Delay  rst=off  infoeditControl=Selection of Reset will increase slice count due to use of real FFs and instead of SRLs  en=off  latency=1  reg_retiming=on  dbl_ovrd=off  block_type=delay
  Delay1 : xbsIndex_r4/Delay  rst=off  infoeditControl=Selection of Reset will increase slice count due to use of real FFs and instead of SRLs  en=off  latency=1  reg_retiming=off  dbl_ovrd=off  block_type=delay
  Delay2 : xbsIndex_r4/Delay  rst=off  infoeditControl=Selection of Reset will increase slice count due to use of real FFs and instead of SRLs  en=off  latency=1  reg_retiming=off  dbl_ovrd=off  block_type=delay
  Delay7 : xbsIndex_r4/Delay  rst=off  infoeditControl=Selection of Reset will increase slice count due to use of real FFs and instead of SRLs  en=off  latency=1  reg_retiming=off  dbl_ovrd=off  block_type=delay
  Inverter : xbsIndex_r4/Inverter  en=off  latency=1  dbl_ovrd=off  block_type=inv
  Inverter1 : xbsIndex_r4/Inverter  en=off  latency=0  dbl_ovrd=off  block_type=inv
  Logical1 : xbsIndex_r4/Logical  logical_function=AND  inputs=2  en=off  latency=1  precision=Full  arith_type=Unsigned  n_bits=8  bin_pt=2  align_bp=on  dbl_ovrd=off  block_type=logical
  Logical2 : xbsIndex_r4/Logical  logical_function=AND  inputs=2  en=off  latency=1  precision=Full  arith_type=Unsigned  n_bits=8  bin_pt=2  align_bp=on  dbl_ovrd=off  block_type=logical
  Logical4 : xbsIndex_r4/Logical  logical_function=OR  inputs=2  en=off  latency=0  precision=Full  arith_type=Unsigned  n_bits=8  bin_pt=2  align_bp=on  dbl_ovrd=off  block_type=logical
  Logical6 : xbsIndex_r4/Logical  logical_function=AND  inputs=3  en=off  latency=0  precision=Full  arith_type=Unsigned  n_bits=8  bin_pt=2  align_bp=on  dbl_ovrd=off  block_type=logical
  Register3 : xbsIndex_r4/Register  init=0  rst=on  en=on  dbl_ovrd=off  block_type=register
  Register4 : xbsIndex_r4/Register  init=0  rst=off  en=on  dbl_ovrd=off  block_type=register
  Register5 : xbsIndex_r4/Register  init=1  rst=on  en=on  dbl_ovrd=off  block_type=register
  Shift : xbsIndex_r4/Shift  shift_dir=Left  shift_bits=32-nsamples-log2(increment)-1-1  en=off  latency=1  precision=Full  arith_type="Signed  (2's comp)"  n_bits=16  bin_pt=14  quantization=Truncate  overflow=Wrap  dbl_ovrd=off  block_type=shift
  add_gen : xbsIndex_r4/Counter  cnt_type=Free Running  cnt_to=1  operation=Up  start_count=0  cnt_by_val=increment  arith_type=Unsigned  n_bits=counter_size  bin_pt=0  load_pin=off  rst=on  en=on  explicit_period=on  period=1  use_behavioral_HDL=off  implementation=DSP48  use_rpm=on  dbl_ovrd=off  block_type=counter
  edge_detect : Subsystem  AncestorBlock=casper_library_misc/edge_detect  mask(edge_detect){edge=Both, polarity=Active High, x_in=[0 0.08 0.08 0.16 0.16 0.24 0.24 0.32 0.32 0.4], y_in=[-1 -1  1  1  1  1 -1 -1 -1 -1], x_out=[0.6 0.68 0.68 0.76 0.76 0.84 0.84 0.92 0.92 1], y_out=[-1 -1  1  1 -1 -1  1  1 -1 -1]}
      mask prompts: edge "Edge Type"; polarity "Output Polarity"; x_in "Input X Positions"; y_in "Input Y Positions"; x_out "Output X Positions"; y_out "Output Y Positions"
      mask help: Output is active for one-cycle after each edge of the specified type (i.e. rising, falling or both).
      mask init:
      | edge_detect_init(gcb,...
      |     'edge',edge,...
      |     'polarity',polarity,...
      |     'x_in',x_in,...
      |     'x_out',x_out,...
      |     'y_in',y_in,...
      |     'y_out',y_out);
      | 
      | x_in_num=str2num(getfield(getfield(get_param(gcb,'UserData'),'parameters'),'x_in'));
      | x_out_num=str2num(getfield(getfield(get_param(gcb,'UserData'),'parameters'),'x_out'));
      | y_in_num=str2num(getfield(getfield(get_param(gcb,'UserData'),'parameters'),'y_in'));
      | y_out_num=str2num(getfield(getfield(get_param(gcb,'UserData'),'parameters'),'y_out'));
  edge_detect1 : Subsystem  AncestorBlock=casper_library_scopes/snapshot/add_gen/edge_detect  mask(edge_detect){edge=Both, polarity=Active High, x_in=[0 0.08 0.08 0.16 0.16 0.24 0.24 0.32 0.32 0.4], y_in=[-1 -1  1  1  1  1 -1 -1 -1 -1], x_out=[0.6 0.68 0.68 0.76 0.76 0.84 0.84 0.92 0.92 1], y_out=[-1 -1  1  1 -1 -1  1  1 -1 -1]}
      mask prompts: edge "Edge Type"; polarity "Output Polarity"; x_in "Input X Positions"; y_in "Input Y Positions"; x_out "Output X Positions"; y_out "Output Y Positions"
      mask help: Output is active for one-cycle after each edge of the specified type (i.e. rising, falling or both).
      mask init:
      | edge_detect_init(gcb,...
      |     'edge',edge,...
      |     'polarity',polarity,...
      |     'x_in',x_in,...
      |     'x_out',x_out,...
      |     'y_in',y_in,...
      |     'y_out',y_out);
      | 
      | x_in_num=str2num(getfield(getfield(get_param(gcb,'UserData'),'parameters'),'x_in'));
      | x_out_num=str2num(getfield(getfield(get_param(gcb,'UserData'),'parameters'),'x_out'));
      | y_in_num=str2num(getfield(getfield(get_param(gcb,'UserData'),'parameters'),'y_in'));
      | y_out_num=str2num(getfield(getfield(get_param(gcb,'UserData'),'parameters'),'y_out'));
  slice1 : xbsIndex_r4/Slice  nbits=nsamples+log2(increment)  boolean_output=off  mode=Lower Bit Location + Width  bit1=0  base1=LSB of Input  bit0=0  base0=LSB of Input  dbl_ovrd=off  block_type=slice
  slice2 : xbsIndex_r4/Slice  nbits=nsamples-burst_size  boolean_output=off  mode=Lower Bit Location + Width  bit1=0  base1=LSB of Input  bit0=log2(increment)+burst_size  base0=LSB of Input  dbl_ovrd=off  block_type=slice
  slice3 : xbsIndex_r4/Slice  nbits=1  boolean_output=on  mode=Lower Bit Location + Width  bit1=0  base1=MSB of Input  bit0=nsamples + log2(increment)  base0=LSB of Input  dbl_ovrd=off  block_type=slice
  vout : Outport
  add : Outport  Port=2
  dout : Outport  Port=3
  we_o : Outport  Port=4
  status : Outport  Port=5
  en_cnt : Outport  Port=6
  done : Outport  Port=7
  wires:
  Delay6/1 -> dout/1
  Delay5/1 -> Delay7/1
  Delay4/1 -> Delay/1, Register3/1, Register3/3, add_gen/1
  Delay3/1 -> Register5/1, Logical4/1
  Delay7/1 -> Register4/1
  Logical1/1 -> Logical6/3
  go/1 -> Logical1/2
  we/1 -> Logical1/1
  Logical4/1 -> Logical6/2
  Inverter/1 -> Concat/2
  slice1/1 -> Delay1/1
  Delay1/1 -> Concat/3
  din/1 -> Delay6/1
  Delay2/1 -> en_cnt/1
  slice2/1 -> add/1
  Convert/1 -> Shift/1
  Concat/1 -> status/1
  Logical6/1 -> add_gen/2, Register3/2, Logical2/1, we_o/1
  init/1 -> Delay4/1
  slice3/1 -> edge_detect/1(in)
  Register5/1 -> Logical6/1, edge_detect1/1(in), Inverter/1, Convert/1
  add_gen/1 -> slice3/1, Delay2/1, slice1/1, slice2/1
  vin/1 -> Delay5/1
  Register3/1 -> Logical2/2
  Logical2/1 -> Register4/2
  Register4/1 -> vout/1
  edge_detect/1(out) -> Register5/3, Inverter1/1
  cont/1 -> Delay3/1
  Inverter1/1 -> Logical4/2
  Delay/1 -> Register5/2
  Shift/1 -> Concat/1
  edge_detect1/1(out) -> done/1
